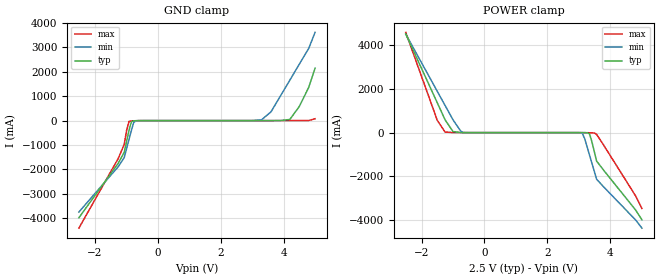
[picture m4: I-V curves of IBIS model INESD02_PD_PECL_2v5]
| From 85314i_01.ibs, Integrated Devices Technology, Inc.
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[Model] INESD02_PD_PECL_2v5
Model_type   Input
Polarity   Non-Inverting
Vinl = 0.8V
Vinh = 2.0V
|   typ   min   max
C_comp   2pF   1.5pF   2.5pF
|   typ   min   max
[Voltage range]  2.5V   2.375V   2.625V
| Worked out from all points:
|   GND clamp passes 1 mA (typ) near -0.59 V on its own axis
|   POWER clamp passes 1 mA (typ) near -0.69 V on its own axis
[GND_clamp]
|Voltage   I(typ)   I(min)   I(max)
-2.5V     -3.983A    -3.749A    -4.408A
-1.25V    -1.747A    -1.889A    -1.551A
-1.061V   -1.3A      -1.517A    -979.1mA
-909.1mV  -407.1mA   -774.3mA   -35.24mA
-833.3mV  -48.47mA   -403.4mA   -14.47mA
-757.6mV  -7.272mA   -70.21mA   -9.677mA
-681.8mV  -2.863mA   -7.067mA   -5.73mA
3.3V      167.2uA    32.81mA    49.66uA
3.6V      586.4uA    357.8mA    70.1uA
4.2V      47.81mA    1.661A     649.6uA
4.8V      1.366A     2.965A     5.596mA
5V        2.15A      3.618A     75.79mA
[POWER_clamp]
|Voltage   I(typ)   I(min)   I(max)
-2.5V     4.503A     4.499A     4.579A
-1.5V     1.366A     1.889A     566.5mA
-1.25V    582.4mA    1.237A     24.21mA
-1V       47.81mA    585.7mA    3.595mA
-681.8mV  586.4uA    6.896mA    416.8uA
3.03V     -323.1uA   -3.378mA   -47.98uA
3.106V    -1.127mA   -30.71mA   -286.5uA
3.182V    -2.863mA   -273.7mA   -1.276mA
3.333V    -48.47mA   -1.016A    -7.036mA
3.561V    -1.3A      -2.13A     -81.94mA
4.8V      -3.536A    -3.991A    -2.894A
5V        -3.983A    -4.363A    -3.465A
